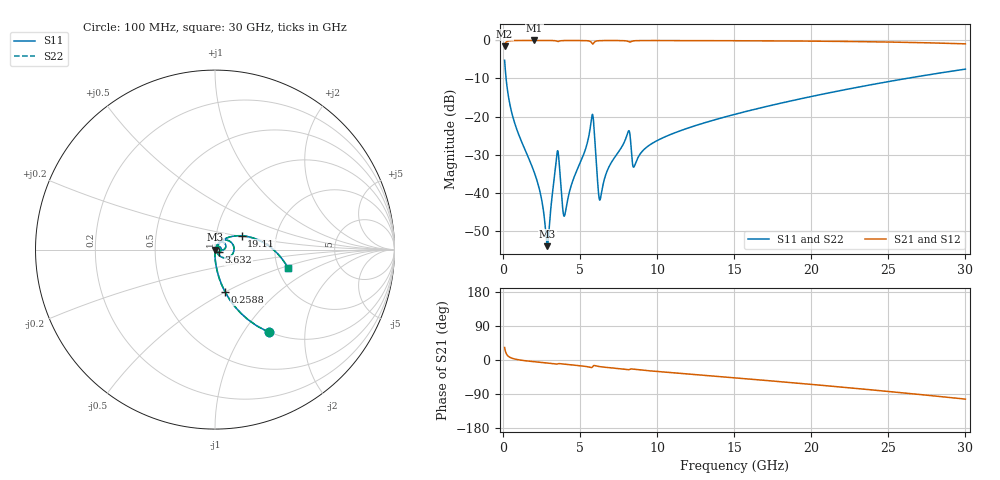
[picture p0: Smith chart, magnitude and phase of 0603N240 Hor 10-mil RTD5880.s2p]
# GHz S MA R 50
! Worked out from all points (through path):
!   3201 points, 100 MHz to 30 GHz, reference 50 ohm
!   highest |S21| = -0.01 dB at 2.034 GHz (marker M1); lowest = -1.6 dB at 100 MHz (marker M2)
!   group delay of S21, straight-line fit = 9.72 ps
!   lowest |S11| = -54.1 dB at 2.875 GHz (marker M3), VSWR 1.00, Z = 50.2 - j0.0404 ohm
!   |S11| at or under -10 dB: 196.3 MHz to 26.18 GHz (25.98 GHz wide, 197 % of centre)
!   |S22| runs from -54.1 to -5.2 dB; largest |S21 - S12| = 0
!   S11 on the Smith chart (normalised r, x): 100 MHz: 0.99, -1.31; 258.8 MHz: 0.99, -0.50; 3.632 GHz: 1.04, -0.03; 19.11 GHz: 1.33, +0.21; 30 GHz: 2.27, -0.56
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0.1  0.5486 -57.0  0.8357 33.0  0.8357 33.0  0.5486 -57.0
0.2588437  0.2444 -76.5  0.9692 13.4  0.9692 13.4  0.2444 -76.5
0.7540625  0.08186 -86.9  0.9959 2.6  0.9959 2.6  0.08186 -86.9
2.034156  0.0182 -90.5  0.9985 -4.6  0.9985 -4.6  0.0182 -90.5
2.875094  0.001977 -11.8  0.998 -8.0  0.998 -8.0  0.001977 -11.8
3.435719  0.0257 41.9  0.9841 -10.7  0.9841 -10.7  0.0257 41.9
3.631937  0.02587 -31.0  0.9758 -9.5  0.9758 -9.5  0.02587 -31.0
3.856187  0.006626 -29.0  0.9937 -10.6  0.9937 -10.6  0.006626 -29.0
3.996344  0.005009 19.0  0.9956 -11.2  0.9956 -11.2  0.005009 19.0
5.089563  0.02701 66.2  0.9957 -15.6  0.9957 -15.6  0.02701 66.2
5.790344  0.1062 9.0  0.9048 -18.9  0.9048 -18.9  0.1062 9.0
5.911812  0.06587 -43.5  0.9418 -14.5  0.9418 -14.5  0.06587 -43.5
6.173438  0.01101 -37.2  0.9896 -16.9  0.9896 -16.9  0.01101 -37.2
6.313594  0.008291 17.2  0.9931 -17.7  0.9931 -17.7  0.008291 17.2
8.088906  0.06105 41.1  0.9741 -25.5  0.9741 -25.5  0.06105 41.1
8.518719  0.02218 35.6  0.9887 -24.6  0.9887 -24.6  0.02218 35.6
10.06978  0.04909 55.6  0.9954 -30.5  0.9954 -30.5  0.04909 55.6
15.05  0.107 40.9  0.9903 -47.1  0.9903 -47.1  0.107 40.9
19.10519  0.1675 27.4  0.9813 -61.2  0.9813 -61.2  0.1675 27.4
20.03956  0.1838 24.1  0.9782 -64.5  0.9782 -64.5  0.1838 24.1
25.01978  0.2879 5.8  0.9519 -83.1  0.9519 -83.1  0.2879 5.8
30  0.4191 -14.0  0.9012 -103.2  0.9012 -103.2  0.4191 -14.0
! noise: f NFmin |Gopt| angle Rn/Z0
0.1  0.0002996  0.9204  0.4072  0.0008323
3.417  0.009943  0.9182  9.472  0.02667
6.743  0.00771  0.8051  18.61  0.008006
10.06  0.008524  0.7472  27.55  0.006405
13.39  0.01009  0.7225  36.32  0.006528
16.7  0.012  0.7134  44.88  0.007087
20.03  0.014  0.7097  53.24  0.007639
23.35  0.0161  0.7097  61.34  0.008157
26.67  0.01836  0.7126  69.24  0.008646
30  0.02082  0.718  76.9  0.009109
